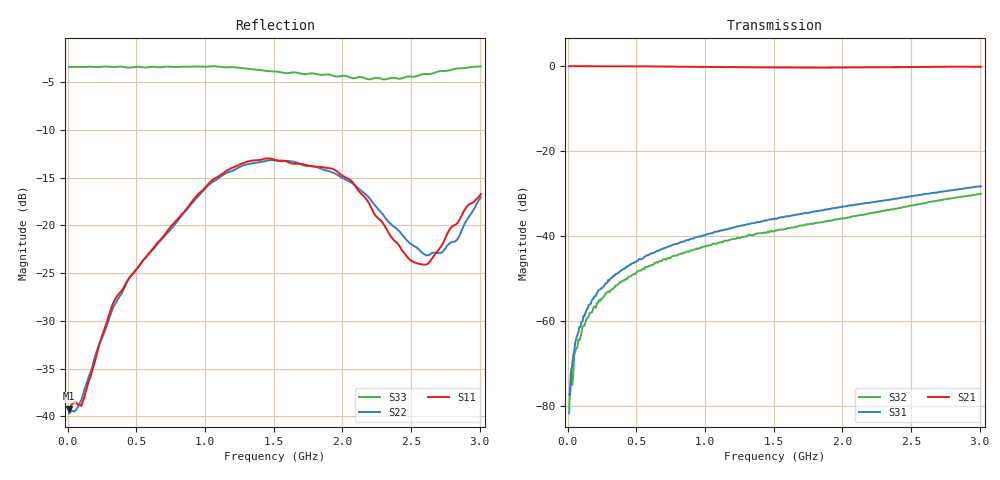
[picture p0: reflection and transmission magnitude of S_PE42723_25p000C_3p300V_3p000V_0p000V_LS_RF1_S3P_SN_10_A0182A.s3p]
! Device ID: PE42723
! File Path: z:\PE42723\Char_75Ohm_20150820\25p000C\3p300\LS_RF1\PE42723_25p000C_3p300V_3p000V_0p000V_LS_RF1_S3P_SN_10_A0182A.s3p
! Serial: 10
! Lot: A0182A
! Temp: 25.000C
! VDD: 3.300
! VSS: 0.000
! Control_Hi: 3.000
! Control_Lo: 0.000
! Logic State: LS_RF1
! Port 1: RFC
! Port 2: RF1
! Port 3: RF2
! ThroughPath:1-2
! IDD: 0.0001149558
! ISS: -1.071e-007
! Comment:
#  Hz  S  RI  R  75
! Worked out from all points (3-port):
!   401 points, 10 MHz to 3.01 GHz, reference 75 ohm
!   strongest paths, dB at 10 MHz, 760 MHz, 1.51 GHz, 2.26 GHz, 3.01 GHz:
!     S21: -0.1, -0.2, -0.4, -0.3, -0.2
!     S31: -77.3, -42.2, -35.9, -31.9, -28.3
!     S32: -81.7, -44.8, -38.9, -34.3, -30.1
!   lowest |S11| = -39.2 dB at 10 MHz (marker M1), VSWR 1.02, Z = 76.7 - j0.0326 ohm
!   |S11| at or under -10 dB: start of sweep to end of sweep
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1e7  0.0109 -0.000213  0.9899 -0.00263  6.97e-05 0.000126
     0.9899 -0.00276  0.0104 -0.000272  9.19e-05 0.000136
     4.02e-06 0.000137  -3.21e-05 7.52e-05  -0.6762 0.00209
5.5e7  0.0117 -0.00188  0.9902 -0.0157  2.43e-05 0.000493
       0.9902 -0.0157  0.0103 -0.0028  -7.07e-06 0.000348
       3.1e-06 0.000561  4.8e-05 0.000434  -0.6777 0.00973
1e8  0.00991 -0.00545  0.9897 -0.029  2.1e-06 0.000947
     0.9898 -0.0289  0.00999 -0.00703  -8.88e-06 0.000682
     -6.13e-06 0.000966  3.41e-05 0.000728  -0.6752 0.0185
3.325e8  0.00877 -0.0383  0.9837 -0.0951  6.34e-05 0.00334
         0.9845 -0.0953  0.00946 -0.0361  8.87e-05 0.0024
         4.43e-05 0.0034  0.000107 0.00242  -0.6735 0.0508
1.03e9  -0.0476 -0.1595  0.9295 -0.2788  0.000881 0.0106
        0.9288 -0.2789  -0.0391 -0.159  0.000425 0.00784
        0.000688 0.0106  0.000462 0.0077  -0.6709 0.1143
1.51e9  -0.0704 -0.209  0.8757 -0.3825  0.00161 0.0159
        0.8762 -0.3825  -0.0647 -0.209  0.000898 0.0115
        0.00162 0.0159  0.000932 0.0114  -0.6237 0.1494
2.0575e9  -0.0739 -0.1567  0.8175 -0.4959  0.00337 0.0223
          0.8175 -0.4965  -0.0578 -0.1586  0.00134 0.0166
          0.00349 0.0225  0.00138 0.0165  -0.5368 0.258
2.5675e9  -0.0373 -0.0504  0.7483 -0.6161  0.0062 0.0298
          0.7493 -0.6142  -0.0124 -0.0727  0.00246 0.0234
          0.0062 0.0297  0.00254 0.0234  -0.4448 0.4239
2.83e9  -0.0745 -0.0688  0.698 -0.6837  0.00893 0.0337
        0.6969 -0.6836  -0.0461 -0.0694  0.00454 0.0278
        0.00879 0.0337  0.00428 0.0278  -0.4489 0.4892
3.01e9  -0.1088 -0.0972  0.6478 -0.7254  0.0113 0.0365
        0.6475 -0.7265  -0.1007 -0.0982  0.00681 0.0305
        0.011 0.0367  0.00678 0.0305  -0.458 0.5047
